(* Logix 5000 Module export ISC_CAM_145; software revision 32.02 *)

MODULES
   ISC_CAM_145 : ETHERNET-MODULE (Ethernet 192.168.1.145, rev 1.1, Output RPI 10 ms)   // isc-camxb145150d
        ISC_CAM_145:I.DATA[0]   // Status
        ISC_CAM_145:I.DATA[0].0   // Life_Bit
        ISC_CAM_145:I.DATA[0].1   // SystemReady
        ISC_CAM_145:I.DATA[0].2   // Belt Moving
        ISC_CAM_145:I.DATA[0].3   // System Error
        ISC_CAM_145:I.DATA[0].4   // System Warning
        ISC_CAM_145:I.DATA[0].5   // System Ready for Next Product
        ISC_CAM_145:I.DATA[0].6   // File reading busy
        ISC_CAM_145:I.DATA[0].7   // Spare
        ISC_CAM_145:I.DATA[0].8   // Spare Byte
        ISC_CAM_145:I.DATA[0].9   // Spare Byte
        ISC_CAM_145:I.DATA[0].10   // Spare Byte
        ISC_CAM_145:I.DATA[0].11   // Spare Byte
        ISC_CAM_145:I.DATA[0].12   // Spare Byte
        ISC_CAM_145:I.DATA[0].13   // Spare Byte
        ISC_CAM_145:I.DATA[0].14   // Spare Byte
        ISC_CAM_145:I.DATA[0].15   // Spare Byte
        ISC_CAM_145:I.DATA[1]   // Fault Code Word 1
        ISC_CAM_145:I.DATA[1].0   // Gap between products to small
        ISC_CAM_145:I.DATA[1].1   // Infeed PE jam
        ISC_CAM_145:I.DATA[1].2   // Outfeed PE jam
        ISC_CAM_145:I.DATA[1].3   // Product buffer too full
        ISC_CAM_145:I.DATA[1].4   // AIM peg sensor fault
        ISC_CAM_145:I.DATA[1].5   // Product destination signal received too late
        ISC_CAM_145:I.DATA[1].8   // Encoder fault
        ISC_CAM_145:I.DATA[1].9   // Motor run signal missing
        ISC_CAM_145:I.DATA[1].10   // Air pressure fault
        ISC_CAM_145:I.DATA[1].12   // IO-Link fault
        ISC_CAM_145:I.DATA[1].13   // Power supply voltage low/high
        ISC_CAM_145:I.DATA[1].15   // Output overcurrent
        ISC_CAM_145:I.DATA[2]   // Fault Code Word 2
        ISC_CAM_145:I.DATA[2].0   // Gap between products to small warning
        ISC_CAM_145:I.DATA[2].1   // Infeed PE jam warning
        ISC_CAM_145:I.DATA[2].2   // Outfeed PE jam warning
        ISC_CAM_145:I.DATA[2].3   // Product buffer nearly full
        ISC_CAM_145:I.DATA[2].4   // AIM damaged or missing peg
        ISC_CAM_145:I.DATA[2].5   // Product destination signal received late
        ISC_CAM_145:I.DATA[2].6   // Product did not sort
        ISC_CAM_145:I.DATA[2].8   // Belt speed too slow
        ISC_CAM_145:I.DATA[2].9   // Belt speed too fast
        ISC_CAM_145:I.DATA[2].10   // Belt elongation limit reached
        ISC_CAM_145:I.DATA[2].11   // Belt acceleration too fast
        ISC_CAM_145:I.DATA[2].12   // Belt deceleration too fast
        ISC_CAM_145:I.DATA[2].14   // High CPU usage
        ISC_CAM_145:I.DATA[3]   // ProductsOnBelt - Count of current products on the belt (Optional in V1 scope)
        ISC_CAM_145:I.DATA[3].0   // IO 0 (C0-Pin4)
        ISC_CAM_145:I.DATA[3].1   // IO 1 (C0-Pin2)
        ISC_CAM_145:I.DATA[3].2   // IO 2 (C1-Pin4)
        ISC_CAM_145:I.DATA[3].3   // IO 3 (C1-Pin2)
        ISC_CAM_145:I.DATA[3].4   // IO 4 (C2-Pin4)
        ISC_CAM_145:I.DATA[3].5   // IO 5 (C2-Pin2)
        ISC_CAM_145:I.DATA[3].6   // IO 6 (C3-Pin4)
        ISC_CAM_145:I.DATA[3].7   // IO 7 (C3-Pin2)
        ISC_CAM_145:I.DATA[3].8   // Spare Byte
        ISC_CAM_145:I.DATA[3].9   // Spare Byte
        ISC_CAM_145:I.DATA[3].10   // Spare Byte
        ISC_CAM_145:I.DATA[3].11   // Spare Byte
        ISC_CAM_145:I.DATA[3].12   // Spare Byte
        ISC_CAM_145:I.DATA[3].13   // Spare Byte
        ISC_CAM_145:I.DATA[3].14   // Spare Byte
        ISC_CAM_145:I.DATA[3].15   // Spare Byte
        ISC_CAM_145:I.DATA[4]   // Split Word - 0-7 Products on Belt Byte, 8-15 Belt Speed Byte
        ISC_CAM_145:I.DATA[4].0   // Products of belt
        ISC_CAM_145:I.DATA[4].1   // Products of belt
        ISC_CAM_145:I.DATA[4].2   // Products of belt
        ISC_CAM_145:I.DATA[4].3   // Products of belt
        ISC_CAM_145:I.DATA[4].4   // Products of belt
        ISC_CAM_145:I.DATA[4].5   // Products of belt
        ISC_CAM_145:I.DATA[4].6   // Products of belt
        ISC_CAM_145:I.DATA[4].7   // Products of belt
        ISC_CAM_145:I.DATA[4].8   // Belt Speed
        ISC_CAM_145:I.DATA[4].9   // Belt Speed
        ISC_CAM_145:I.DATA[4].10   // Belt Speed
        ISC_CAM_145:I.DATA[4].11   // Belt Speed
        ISC_CAM_145:I.DATA[4].12   // Belt Speed
        ISC_CAM_145:I.DATA[4].13   // Belt Speed
        ISC_CAM_145:I.DATA[4].14   // Belt Speed
        ISC_CAM_145:I.DATA[4].15   // Belt Speed
        ISC_CAM_145:I.DATA[5]   // Throughput - number of product inducted per minute
        ISC_CAM_145:I.DATA[6]   // Destination last product Byte - bits 0-7
        ISC_CAM_145:I.DATA[6].0   // Destination last product
        ISC_CAM_145:I.DATA[6].1   // Destination last product
        ISC_CAM_145:I.DATA[6].2   // Destination last product
        ISC_CAM_145:I.DATA[6].3   // Destination last product
        ISC_CAM_145:I.DATA[6].4   // Destination last product
        ISC_CAM_145:I.DATA[6].5   // Destination last product
        ISC_CAM_145:I.DATA[6].6   // Destination last product
        ISC_CAM_145:I.DATA[6].7   // Destination last product
        ISC_CAM_145:I.DATA[6].8   // Spare byte
        ISC_CAM_145:I.DATA[6].9   // Spare byte
        ISC_CAM_145:I.DATA[6].10   // Spare byte
        ISC_CAM_145:I.DATA[6].11   // Spare byte
        ISC_CAM_145:I.DATA[6].12   // Spare byte
        ISC_CAM_145:I.DATA[6].13   // Spare byte
        ISC_CAM_145:I.DATA[6].14   // Spare byte
        ISC_CAM_145:I.DATA[6].15   // Spare byte
        ISC_CAM_145:I.DATA[7]   // Spare Word
        ISC_CAM_145:I.DATA[8]   // Spare Word
        ISC_CAM_145:I.DATA[9]   // Spare Word
        ISC_CAM_145:I.DATA[10]   // Spare Word
        ISC_CAM_145:I.DATA[11]   // Spare Word
        ISC_CAM_145:I.DATA[12]   // Parameter group 1 byte - bits 0-7, Paramet feedback 1 byte - 8-15
        ISC_CAM_145:I.DATA[12].0   // Parameter group
        ISC_CAM_145:I.DATA[12].1   // Parameter group
        ISC_CAM_145:I.DATA[12].2   // Parameter group
        ISC_CAM_145:I.DATA[12].3   // Parameter group
        ISC_CAM_145:I.DATA[12].4   // Parameter group
        ISC_CAM_145:I.DATA[12].5   // Parameter group
        ISC_CAM_145:I.DATA[12].6   // Parameter group
        ISC_CAM_145:I.DATA[12].7   // Parameter group
        ISC_CAM_145:I.DATA[12].8   // Parameter read OK
        ISC_CAM_145:I.DATA[12].9   // Parameter write OK
        ISC_CAM_145:I.DATA[12].10   // Parameter type OK
        ISC_CAM_145:I.DATA[12].11   // Parameter value format OK
        ISC_CAM_145:I.DATA[12].12   // Spare bit
        ISC_CAM_145:I.DATA[12].13   // Spare bit
        ISC_CAM_145:I.DATA[12].14   // Spare bit
        ISC_CAM_145:I.DATA[12].15   // Spare bit
        ISC_CAM_145:I.DATA[13]   // Parameter
        ISC_CAM_145:I.DATA[14]   // Parameter value LSW
        ISC_CAM_145:I.DATA[15]   // Parameter value MSW
        ISC_CAM_145:O.DATA[0]   // Status
        ISC_CAM_145:O.DATA[0].0   // Life_Bit
        ISC_CAM_145:O.DATA[0].1   // Belt motor running
        ISC_CAM_145:O.DATA[0].3   // Reset errors
        ISC_CAM_145:O.DATA[0].4   // Reset warnings
        ISC_CAM_145:O.DATA[0].5   // Reset destination counter
        ISC_CAM_145:O.DATA[0].9   // Reserved - set always as 0
        ISC_CAM_145:O.DATA[0].12   // Product from infeed 1
        ISC_CAM_145:O.DATA[0].13   // Product from infeed 2
        ISC_CAM_145:O.DATA[1]   // Product destination 1 Byte - bits 0-7 - Run modes 1 Byet - bits 8-15
        ISC_CAM_145:O.DATA[1].0   // Product destination
        ISC_CAM_145:O.DATA[1].1   // Product destination
        ISC_CAM_145:O.DATA[1].2   // Product destination
        ISC_CAM_145:O.DATA[1].3   // Product destination
        ISC_CAM_145:O.DATA[1].4   // Product destination
        ISC_CAM_145:O.DATA[1].5   // Product destination
        ISC_CAM_145:O.DATA[1].6   // Product destination
        ISC_CAM_145:O.DATA[1].7   // Product destination
        ISC_CAM_145:O.DATA[1].8   // Run mode internal
        ISC_CAM_145:O.DATA[1].9   // Run mode PLC
        ISC_CAM_145:O.DATA[1].15   // Reserved - set always as 0
        ISC_CAM_145:O.DATA[2]   // Spare word
        ISC_CAM_145:O.DATA[3]   // Destination 0 1 Byte - bits 0-7, Destination 1 1 Byte - bits 8 15
        ISC_CAM_145:O.DATA[3].0   // Destination 0
        ISC_CAM_145:O.DATA[3].1   // Destination 0
        ISC_CAM_145:O.DATA[3].2   // Destination 0
        ISC_CAM_145:O.DATA[3].3   // Destination 0
        ISC_CAM_145:O.DATA[3].4   // Destination 0
        ISC_CAM_145:O.DATA[3].5   // Destination 0
        ISC_CAM_145:O.DATA[3].6   // Destination 0
        ISC_CAM_145:O.DATA[3].7   // Destination 0
        ISC_CAM_145:O.DATA[3].8   // Destination 1
        ISC_CAM_145:O.DATA[3].9   // Destination 1
        ISC_CAM_145:O.DATA[3].10   // Destination 1
        ISC_CAM_145:O.DATA[3].11   // Destination 1
        ISC_CAM_145:O.DATA[3].12   // Destination 1
        ISC_CAM_145:O.DATA[3].13   // Destination 1
        ISC_CAM_145:O.DATA[3].14   // Destination 1
        ISC_CAM_145:O.DATA[3].15   // Destination 1
        ISC_CAM_145:O.DATA[4]   // Destination 2 1 Byte - bits 0-7, Destination 3 1 Byte - bits 8 15
        ISC_CAM_145:O.DATA[4].0   // Destination 2
        ISC_CAM_145:O.DATA[4].1   // Destination 2
        ISC_CAM_145:O.DATA[4].2   // Destination 2
        ISC_CAM_145:O.DATA[4].3   // Destination 2
        ISC_CAM_145:O.DATA[4].4   // Destination 2
        ISC_CAM_145:O.DATA[4].5   // Destination 2
        ISC_CAM_145:O.DATA[4].6   // Destination 2
        ISC_CAM_145:O.DATA[4].7   // Destination 2
        ISC_CAM_145:O.DATA[4].8   // Destination 3
        ISC_CAM_145:O.DATA[4].9   // Destination 3
        ISC_CAM_145:O.DATA[4].10   // Destination 3
        ISC_CAM_145:O.DATA[4].11   // Destination 3
        ISC_CAM_145:O.DATA[4].12   // Destination 3
        ISC_CAM_145:O.DATA[4].13   // Destination 3
        ISC_CAM_145:O.DATA[4].14   // Destination 3
        ISC_CAM_145:O.DATA[4].15   // Destination 3
        ISC_CAM_145:O.DATA[5]   // Destination 4 1 Byte - bits 0-7, Destination 5 1 Byte - bits 8 15
        ISC_CAM_145:O.DATA[5].0   // Destination 4
        ISC_CAM_145:O.DATA[5].1   // Destination 4
        ISC_CAM_145:O.DATA[5].2   // Destination 4
        ISC_CAM_145:O.DATA[5].3   // Destination 4
        ISC_CAM_145:O.DATA[5].4   // Destination 4
        ISC_CAM_145:O.DATA[5].5   // Destination 4
        ISC_CAM_145:O.DATA[5].6   // Destination 4
        ISC_CAM_145:O.DATA[5].7   // Destination 4
        ISC_CAM_145:O.DATA[5].8   // Destination 5
        ISC_CAM_145:O.DATA[5].9   // Destination 5
        ISC_CAM_145:O.DATA[5].10   // Destination 5
        ISC_CAM_145:O.DATA[5].11   // Destination 5
        ISC_CAM_145:O.DATA[5].12   // Destination 5
        ISC_CAM_145:O.DATA[5].13   // Destination 5
        ISC_CAM_145:O.DATA[5].14   // Destination 5
        ISC_CAM_145:O.DATA[5].15   // Destination 5
        ISC_CAM_145:O.DATA[6]   // Destination 6 1 Byte - bits 0-7, Reserved set 0 1 Byte - bits 8 15
        ISC_CAM_145:O.DATA[6].0   // Destination 6
        ISC_CAM_145:O.DATA[6].1   // Destination 6
        ISC_CAM_145:O.DATA[6].2   // Destination 6
        ISC_CAM_145:O.DATA[6].3   // Destination 6
        ISC_CAM_145:O.DATA[6].4   // Destination 6
        ISC_CAM_145:O.DATA[6].5   // Destination 6
        ISC_CAM_145:O.DATA[6].6   // Destination 6
        ISC_CAM_145:O.DATA[6].7   // Destination 6
        ISC_CAM_145:O.DATA[6].8   // Reserved - set 0
        ISC_CAM_145:O.DATA[6].9   // Reserved - set 0
        ISC_CAM_145:O.DATA[6].10   // Reserved - set 0
        ISC_CAM_145:O.DATA[6].11   // Reserved - set 0
        ISC_CAM_145:O.DATA[6].12   // Reserved - set 0
        ISC_CAM_145:O.DATA[6].13   // Reserved - set 0
        ISC_CAM_145:O.DATA[6].14   // Reserved - set 0
        ISC_CAM_145:O.DATA[6].15   // Reserved - set 0
        ISC_CAM_145:O.DATA[7]   // Carryway enable 1 byte - bits 0-7 Override active carryway pointer 1 byte - bits 8-15
        ISC_CAM_145:O.DATA[7].0   // Reserved
        ISC_CAM_145:O.DATA[7].1   // Reserved
        ISC_CAM_145:O.DATA[7].2   // Active carryway 1 enable left
        ISC_CAM_145:O.DATA[7].3   // Active carryway 1 enable right
        ISC_CAM_145:O.DATA[7].4   // Active carryway 2 enable left
        ISC_CAM_145:O.DATA[7].5   // Active carryway 2 enable right
        ISC_CAM_145:O.DATA[7].6   // Active carryway 3 enable left
        ISC_CAM_145:O.DATA[7].7   // Active carryway 3 enable right
        ISC_CAM_145:O.DATA[7].8   // Override active carryway pointer
        ISC_CAM_145:O.DATA[7].9   // Override active carryway pointer
        ISC_CAM_145:O.DATA[7].10   // Override active carryway pointer
        ISC_CAM_145:O.DATA[7].11   // Override active carryway pointer
        ISC_CAM_145:O.DATA[7].12   // Override active carryway pointer
        ISC_CAM_145:O.DATA[7].13   // Override active carryway pointer
        ISC_CAM_145:O.DATA[7].14   // Override active carryway pointer
        ISC_CAM_145:O.DATA[7].15   // Override active carryway pointer
        ISC_CAM_145:O.DATA[8]   // Carryway control
        ISC_CAM_145:O.DATA[8].1   // Active carryway 1 enable
        ISC_CAM_145:O.DATA[8].2   // Active carryway 2 enable
        ISC_CAM_145:O.DATA[8].3   // Active carryway 3 enable
        ISC_CAM_145:O.DATA[8].9   // Override active carryway 1
        ISC_CAM_145:O.DATA[8].10   // Override active carryway 2
        ISC_CAM_145:O.DATA[8].11   // Override active carryway 3
        ISC_CAM_145:O.DATA[9]   // Override active carryway value
        ISC_CAM_145:O.DATA[10]   // Spare word
        ISC_CAM_145:O.DATA[11]   // Spare word
        ISC_CAM_145:O.DATA[12]   // Parameter group 1 byte - bits 0-7 Parameter R/W 1 byte - bits 8-15
        ISC_CAM_145:O.DATA[12].0   // Parameter group
        ISC_CAM_145:O.DATA[12].1   // Parameter group
        ISC_CAM_145:O.DATA[12].2   // Parameter group
        ISC_CAM_145:O.DATA[12].3   // Parameter group
        ISC_CAM_145:O.DATA[12].4   // Parameter group
        ISC_CAM_145:O.DATA[12].5   // Parameter group
        ISC_CAM_145:O.DATA[12].6   // Parameter group
        ISC_CAM_145:O.DATA[12].7   // Parameter group
        ISC_CAM_145:O.DATA[12].8   // Parameter read value
        ISC_CAM_145:O.DATA[12].9   // Parameter write value
        ISC_CAM_145:O.DATA[12].10   // Spare bit
        ISC_CAM_145:O.DATA[12].11   // Spare bit
        ISC_CAM_145:O.DATA[12].12   // Spare bit
        ISC_CAM_145:O.DATA[12].13   // Spare bit
        ISC_CAM_145:O.DATA[12].14   // Spare bit
        ISC_CAM_145:O.DATA[12].15   // Spare bit
        ISC_CAM_145:O.DATA[13]   // Parameter
        ISC_CAM_145:O.DATA[13].0   // Read Parameter
        ISC_CAM_145:O.DATA[13].1   // Whrite Parameter
        ISC_CAM_145:O.DATA[14]   // Parameter value
        ISC_CAM_145:O.DATA[15]   // Spare Word
END_MODULES
